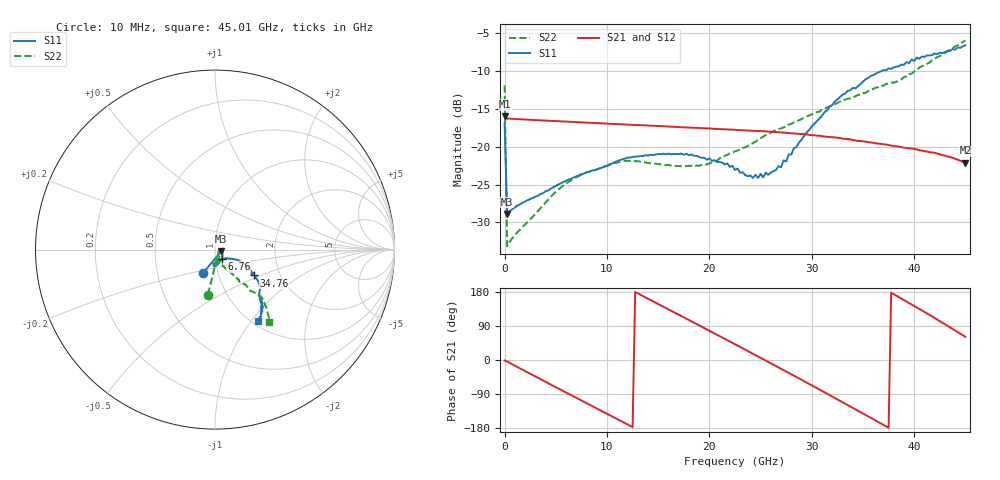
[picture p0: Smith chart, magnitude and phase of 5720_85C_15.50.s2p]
! Device:  ADRF5720
! Description: 0.5dB LSB GaAs MMIC 6-bit Digital Attenuator
! Frequency:  0.000009 -  40 GHz
! Ports:
!	RF1	= Port 1
!	RF2	= Port 2
! Vdd:  3.3 Volt
! Vss:  -3.3 Volt
! Control:  0/3.3 Volt
! State:  15.50 dB attenuation
! Data:  The device was measured using G-S-G Probes on a matrix board.
!  Data was collected using an calibrated 4 port network analyzer.
!  The reference plane for this measurement is at the launchers.
! Note:  Analog Devices supplies this data as a sample of measured data
!  for this product.  Your particular data for this product may vary.
!  Data was taken at 85 degrees C.
!  Analog Devices reserves the right to change this data at anytime.
# GHZ S DB R 45.0
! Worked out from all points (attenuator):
!   181 points, 10 MHz to 45.01 GHz, reference 45 ohm
!   highest |S21| = -15.98 dB at 10 MHz (marker M1); lowest = -22.1 dB at 45.01 GHz (marker M2)
!   lowest |S11| = -28.9 dB at 260 MHz (marker M3), VSWR 1.07, Z = 48.2 - j0.821 ohm
!   |S11| at or under -10 dB: start of sweep to 36.82 GHz
!   |S22| runs from -33.1 to -6.0 dB; largest |S21 - S12| = 0.00083
!   S11 on the Smith chart (normalised r, x): 10 MHz: 0.85, -0.22; 6.76 GHz: 1.07, -0.11; 34.76 GHz: 1.47, -0.45; 45.01 GHz: 1.06, -1.09
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0.01  -16.89 -116.7  -15.98 -1.5  -15.97 -1.5  -11.91 -98.9
0.26  -28.89 -13.7  -16.27 -4.0  -16.26 -3.9  -33.13 -21.7
3.76  -26.14 -31.9  -16.52 -54.1  -16.51 -54.1  -27.78 -52.0
6.76  -24.05 -54.2  -16.72 -96.4  -16.71 -96.3  -24.22 -75.4
7.76  -23.54 -59.6  -16.79 -110.4  -16.78 -110.3  -23.54 -80.1
11.51  -21.65 -77.8  -17.04 -163.0  -17.03 -162.9  -21.91 -93.8
15.26  -20.98 -89.7  -17.27 144.2  -17.26 144.3  -22.32 -96.2
19.51  -21.46 -94.9  -17.56 84.2  -17.54 84.4  -22.43 -80.1
22.76  -22.87 -85.8  -17.78 38.0  -17.77 38.3  -20.49 -66.4
24.76  -24.12 -70.4  -17.92 9.5  -17.91 9.8  -19.11 -62.0
27.01  -22.71 -42.0  -18.10 -23.1  -18.08 -22.9  -17.56 -56.9
27.26  -21.79 -38.5  -18.13 -26.8  -18.12 -26.6  -17.42 -57.2
27.51  -21.96 -37.2  -18.17 -30.4  -18.15 -30.1  -17.31 -56.1
27.76  -21.01 -34.2  -18.19 -34.0  -18.18 -33.7  -17.08 -56.9
28.01  -21.03 -34.2  -18.23 -37.7  -18.21 -37.4  -16.98 -56.2
30.26  -16.97 -26.2  -18.49 -70.5  -18.48 -70.3  -15.67 -54.7
33.01  -13.13 -29.0  -18.92 -111.4  -18.90 -111.1  -13.88 -52.7
34.76  -11.71 -33.6  -19.24 -137.3  -19.22 -137.0  -13.15 -52.6
37.76  -9.71 -40.5  -19.85 177.4  -19.83 177.7  -11.53 -49.0
41.51  -7.93 -49.7  -20.72 119.0  -20.69 119.3  -8.87 -45.7
43.51  -7.36 -52.0  -21.37 86.3  -21.34 86.7  -7.13 -49.1
45.01  -6.61 -58.8  -22.10 61.1  -22.07 61.5  -5.96 -53.4
